(* Logix 5000 AddOnInstructionDefinition export T2JOG; software revision 32.02 *)

TYPE Exlar_Control :   // Tritex II Control
STRUCT
   EnableOutputs : INT;   // EnableOutputs
   InputEventsMode : INT;   // 4316
   InputEventsModeLevel : INT;   // 4318
   InputEventsMotion : INT;   // 4317
   HostCommandControlMode : INT;   // 4303
   HostPosition_low : INT;   // 4304
   HostPosition_high : INT;
   HostVelocity_low : INT;   // 4306
   HostVelocity_high : INT;
   HostAcceleration_low : INT;   // 4308
   HostAcceleration_high : INT;
   HostCurrent : INT;   // 4310
   InputEventsMoveEdge : INT;   // 4319
   JogSlowVelocity_low : INT;   // 6022
   JogSlowVelocity_high : INT;
   JogAcceleration_low : INT;   // 6026
   JogAcceleration_high : INT;
   MoveOption : INT;   // 6100
   MoveCurrentLimit : INT;   // 6101
   MoveAcceleration_low : INT;   // 6102
   MoveAcceleration_high : INT;
   MoveDeceleration_low : INT;   // 6500
   MoveDeceleration_high : INT;
   MovePrimaryOption : INT;   // 6106
   spare : INT;   // spare
   MovePrimaryPosition_low : INT;   // 6108
   MovePrimaryPosition_high : INT;
   MovePrimaryVelocity_low : INT;   // 6110
   MovePrimaryVelocity_high : INT;
   MoveSecondaryOption : INT;   // 6112
   spare2 : INT;   // spare
   MoveSecondaryPosition_low : INT;   // 6114
   MoveSecondaryPosition_high : INT;
   MoveSecondaryVelocity_low : INT;   // 6116
   MoveSecondaryVelocity_high : INT;
END_STRUCT
END_TYPE

TYPE Exlar_Drive :   // Tritex II Data
STRUCT
   Control : Exlar_Control;   // Control bits to send to the drive
   Status : Exlar_Status;   // Status bits received from the drive
END_STRUCT
END_TYPE

TYPE Exlar_Status :   // Tritex II Status
STRUCT
   EIP_Comm : INT;   // EIP module communication
   OutputEventsStatus : INT;   // 104
   OutputEventsMoveInPosition : INT;   // 108
   OutputEventsMotion : INT;   // 105
   OutputsEventsMotionActive : INT;   // 107
   PositionFeedback_low : INT;   // 378
   PositionFeedback_high : INT;
   SoftFaults : INT;   // 7
   HardFaults : INT;   // 6
   VelocityDisplay_low : INT;   // 356
   VelocityDisplay_high : INT;
   CurrentDisplay : INT;   // 567
   CurrentContinuous : INT;   // 565
   CurrentLimit : INT;   // 5108
   VoltageHallBattery : INT;   // 8
   VoltageBus : INT;   // 571
   TemperatureBoard : INT;   // 11
   TemperatureActuator : INT;   // 15
END_STRUCT
END_TYPE

ADD_ON_INSTRUCTION T2JOG   (* revision 1.1, vendor Exlar Corporation *)
// Help:
// Use the Tritex 2 Jog (T2JOG) instruction to move an a drive at a constant speed until you tell it to stop.
// Jog commands includes enabling Jog Positive or Negative.  The instruction allow user to select profile velocity and acceleration in user units.
// Configured for Exlar EIP AOI. 07/01/2014
// ----------------------------------------------------------------------------------------------------------------------------
// Parameters Bit Definition
// ----------------------------------------------------------------------------------------------------------------------------
// Direction:  (Input) Command Jog Direction
// ------------------------------------------------------------------
//      Direction.0:     Jog Plus
//      Direction.1:     Jog Minus
// Active:  (Output) Jog status information
// ------------------------------------------------------------------
//      Active.0:     Jog Plus active
//      Active.1:     Jog Minus active
//      Active.2:     Ready
VAR_IN_OUT
   Drive : Exlar_Drive; {required}   // Drive
   Units : REAL[5]; {required}   // User Units Configuration
END_VAR
VAR_INPUT
   Direction : INT; {access Read Only, visible}   // Jog Control
        .0   // JOGP
        .1   // JOGN
   Velocity : REAL; {access Read Only, visible}   // Speed to move the drive in Speed Units.
   Acceleration : REAL; {access Read Only, visible}   // Acceleration rate of the drive in Accel Units.
END_VAR
VAR_OUTPUT
   DF : BOOL; {access Read Only, visible}   // A Drive Fault is active
   ER : BOOL; {access Read Only, visible}   // A Instruction error is Active
   Active : INT; {access Read Only, visible}   // Jog Active States
        .0   // JOGP
        .1   // JOGN
        .2   // STOPPED
        .3   // READY
END_VAR
VAR
   tempDINT : DINT; {access None}   // Temporary Register used in calculating units
END_VAR

ROUTINE Logic   (* structured text *)
   (***********************************************)
   (*   Exlar Tritex 2 Jog                        *)
   (*                                             *)
   (***********************************************)
   
   
   
   (*********** INPUTS ***********)
   
   (* Direction *)
   	(* 4317.4 Jog Positive *)
   	If Direction.0 Then
   		Drive.Control.InputEventsMotion.4 := 1;
   	else
   		Drive.Control.InputEventsMotion.4 := 0;
   	end_if;
   
   	(* 4317.5 Jog Minus *)
   	If Direction.1 Then
   		Drive.Control.InputEventsMotion.5 := 1;
   	else
   		Drive.Control.InputEventsMotion.5 := 0;
   	end_if;
   
   (*********** OUTPUTS  ***********)
   
   (* Drive Faults Active *)
   	(* 104.03 Fault *)
   	If Drive.Status.OutputEventsStatus.3 then
    		DF := 1;
   	Else
   		DF := 0;
   	End_If;
   
   (* Active States  *)
   	(* 105.3 JOG Positive *)
   	If Drive.Status.OutputEventsMotion.3 Then
   		Active.0 := 1;
   	else
   		Active.0 := 0;
   	end_if;
   
   	(* 105.4 JOG Minus *)
   	If Drive.Status.OutputEventsMotion.4 Then
   		Active.1 := 1;
   	else
   		Active.1 := 0;
   	end_if;
   
   
   	(* 105.0 STOPPED *)
   	If Drive.Status.OutputEventsMotion.0 Then
   		Active.2 := 1;
   	else
   		Active.2 := 0;
   	end_if;
   
   	(* 104.2 Ready *)
   	If Drive.Status.OutputEventsStatus.2 Then
   		Active.3 := 1;
   	else
   		Active.3 := 0;
   	end_if;
   
   
   (* Convert Units *)
   	IF Units[0] = 0 THEN
   		ER	:= 1;
   	else
   		ER  := 0;
   
   		(* Jog.SlowVelovity : ModuleOutputs[14],ModuleOutputs[13] *)
   		tempDINT := Velocity / Units[2];
   		cps(tempDINT, Drive.Control.JogSlowVelocity_low,2);
   
   		(* Jog.Acceleration: ModuleOutputs[16],ModuleOutputs[15] *)
   		tempDINT := Acceleration / Units[3];
   		cps(tempDINT, Drive.Control.JogAcceleration_low,2);
   
   	end_if;
END_ROUTINE
END_ADD_ON_INSTRUCTION
